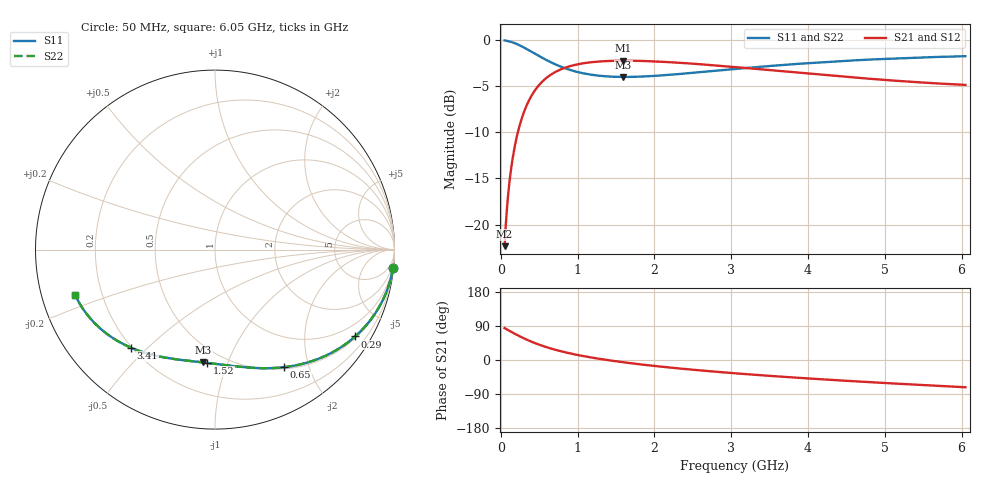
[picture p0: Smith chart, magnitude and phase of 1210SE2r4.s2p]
! AVX Thin Film Operation		Date: August 2001
! Description: Accu-P® Series, Thin Film, SMD, RF Capacitor
! Part Number: 12101J2R4ABT
! 50 MHz  -  6.05 GHz
! Serial Measurements
# mhz S db R 50
!	S11		S21		S12		S22
!	dB	Phase	dB	Phase	dB	Phase	dB	Phase
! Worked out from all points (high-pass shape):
!   401 points, 50 MHz to 6.05 GHz, reference 50 ohm
!   highest |S21| = -2.22 dB at 1.595 GHz (marker M1); lowest = -22.3 dB at 50 MHz (marker M2)
!   |S21| within 3 dB of the highest: 464.3 MHz to end of sweep
!   lowest |S11| = -4.0 dB at 1.595 GHz (marker M3), VSWR 4.44, Z = 19.6 - j41.1 ohm
!   |S11| at or under -10 dB: nowhere
!   |S22| runs from -4.0 to 0.0 dB; largest |S21 - S12| = 0
!   S11 on the Smith chart (normalised r, x): 50 MHz: 1, -20; 290 MHz: 0.55, -3.43; 650 MHz: 0.52, -1.62; 1.52 GHz: 0.40, -0.85; 3.41 GHz: 0.20, -0.45; 6.05 GHz: 0.10, -0.16
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50  -0.03 -5.8  -22.34 84.2  -22.34 84.2  -0.03 -5.8
65  -0.04 -7.6  -20.09 82.4  -20.09 82.4  -0.04 -7.6
110  -0.12 -12.8  -15.62 77.2  -15.62 77.2  -0.12 -12.8
155  -0.23 -17.8  -12.80 72.2  -12.80 72.2  -0.23 -17.8
215  -0.43 -24.3  -10.23 65.7  -10.23 65.7  -0.43 -24.3
290  -0.74 -31.8  -8.06 58.2  -8.06 58.2  -0.74 -31.8
365  -1.08 -38.7  -6.57 51.3  -6.57 51.3  -1.08 -38.7
455  -1.51 -46.2  -5.32 43.8  -5.32 43.8  -1.51 -46.2
545  -1.93 -52.8  -4.45 37.2  -4.45 37.2  -1.93 -52.8
650  -2.38 -59.5  -3.75 30.5  -3.75 30.5  -2.38 -59.5
845  -3.06 -69.9  -2.96 20.1  -2.96 20.1  -3.06 -69.9
1055  -3.56 -78.9  -2.53 11.1  -2.53 11.1  -3.56 -78.9
1265  -3.84 -86.3  -2.32 3.7  -2.32 3.7  -3.84 -86.3
1520  -3.98 -93.9  -2.22 -3.9  -2.22 -3.9  -3.98 -93.9
1595  -3.98 -95.9  -2.22 -6.0  -2.22 -6.0  -3.98 -95.9
2060  -3.84 -106.9  -2.32 -17.0  -2.32 -17.0  -3.84 -106.9
2525  -3.52 -116.1  -2.56 -26.1  -2.56 -26.1  -3.52 -116.1
3050  -3.12 -125.0  -2.91 -35.1  -2.91 -35.1  -3.12 -125.0
3410  -2.86 -130.5  -3.17 -40.5  -3.17 -40.5  -2.86 -130.5
4055  -2.46 -139.3  -3.66 -49.4  -3.66 -49.4  -2.46 -139.3
5060  -2.00 -151.3  -4.34 -61.4  -4.34 -61.4  -2.00 -151.3
6050  -1.74 -161.8  -4.85 -71.9  -4.85 -71.9  -1.74 -161.9
